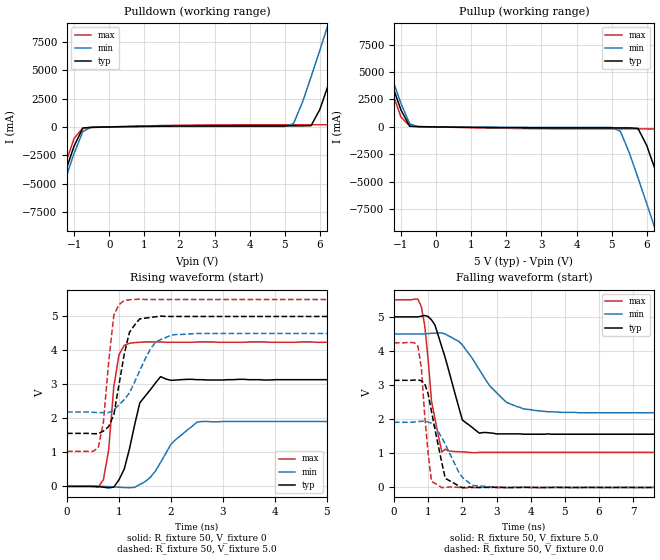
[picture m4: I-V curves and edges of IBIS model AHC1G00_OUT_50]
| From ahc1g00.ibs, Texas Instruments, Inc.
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|   Model AHC1G00_OUT_50
[Model]   AHC1G00_OUT_50
Model_type  Output
Polarity   Inverting
Vmeas = 2.50v
Cref = 15pf
| variable   typ   min   max
C_comp   3.12pf   2.34pf   3.90pf
[Temperature Range]   25   85   -40
[Voltage Range]   5.0   4.5   5.5
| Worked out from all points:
|   slope of the pulldown table from 0 to 0.75 V, typ, clamps not added: 18.8 ohm
|   slope of the pullup table from 0 to 0.75 V, typ, clamps not added: 25.3 ohm
|   rising waveform, R_fixture 50, V_fixture 0: 20-80 % time 307ps typ, 550ps min, 174ps max; typ from 0 V to 3.14 V
|   falling waveform, R_fixture 50, V_fixture 5.0: 20-80 % time 586ps typ, 1.03ns min, 304ps max; typ from 5 V to 1.56 V
|   rising waveform, R_fixture 50, V_fixture 5.0: 20-80 % time 250ps typ, 453ps min, 167ps max; typ from 1.56 V to 5 V
|   falling waveform, R_fixture 50, V_fixture 0.0: 20-80 % time 378ps typ, 581ps min, 209ps max; typ from 3.14 V to 0 V
[Pulldown]
|   Voltage   I(typ)   I(min)   I(max)
-5V       -40.9A     -41.4A     -40.3A
-1.75V    -8.76A     -9.39A     -8.09A
-1V       -1.69A     -2.33A     -1.02A
-750mV    -95.5mA    -395mA     -80.6mA
5.25V     93.4mA     298mA      192mA
5.75V     116mA      4.42A      192mA
6.25V     3.8A       9.19A      193mA
6.5V      6.17A      11.6A      931mA
6.75V     8.59A      14.1A      3.15A
7.25V     13.5A      19A        7.96A
7.5V      15.9A      21.4A      10.4A
10V       40.7A      46.2A      35.2A
[Pullup]
|   Voltage   I(typ)   I(min)   I(max)
-5V       40.7A      41.2A      40.1A
-2V       11A        11.6A      10.4A
-1.75V    8.59A      9.19A      7.96A
-1V       1.54A      2.14A      907mA
-750mV    63.6mA     284mA      62.5mA
5.25V     -84.4mA    -401mA     -178mA
5.75V     -130mA     -4.62A     -178mA
6.25V     -3.97A     -9.39A     -187mA
6.75V     -8.76A     -14.3A     -3.28A
7.25V     -13.6A     -19.2A     -8.09A
7.5V      -16.1A     -21.6A     -10.5A
10V       -40.9A     -46.4A     -35.3A
[Ramp]
| variable   typ   min   max
dV/dt_r   1.90E+00/3.24E-10   1.17E+00/4.90E-10   2.56E+00/1.49E-10
dV/dt_f   2.09E+00/5.17E-10   1.41E+00/1.00E-09   2.74E+00/2.95E-10
R_load = 50
[Rising Waveform]
R_fixture = 50
V_fixture = 0
|   Time   V(typ)   V(min)   V(max)
0s        0V         0V         0V
700ps     -23.1mV    -236uV     201mV
800ps     -43.2mV    -5.91mV    1.07V
900ps     -22.1mV    -13.9mV    2.94V
1ns       197mV      -24.2mV    3.88V
1.3ns     1.81V      -28.1mV    4.23V
1.4ns     2.46V      55.2mV     4.24V
1.8ns     3.23V      706mV      4.25V
2.6ns     3.14V      1.91V      4.25V
25ns      3.14V      1.91V      4.24V
[Falling Waveform]
R_fixture = 50
V_fixture = 5.0
V_fixture_min = 4.5
V_fixture_max = 5.5
|   Time   V(typ)   V(min)   V(max)
0s        5V         4.5V       5.5V
800ps     5.02V      4.5V       5.3V
900ps     5.04V      4.5V       4.75V
1.1ns     4.91V      4.52V      2.52V
1.4ns     4.12V      4.53V      1.04V
2ns       1.98V      4.18V      1.04V
2.5ns     1.59V      3.45V      1.03V
3.3ns     1.57V      2.49V      1.03V
4.5ns     1.57V      2.22V      1.03V
25ns      1.56V      2.19V      1.03V
[Rising Waveform]
R_fixture = 50
V_fixture = 5.0
V_fixture_min = 4.5
V_fixture_max = 5.5
|   Time   V(typ)   V(min)   V(max)
0s        1.56V      2.19V      1.03V
600ps     1.55V      2.17V      1.14V
700ps     1.63V      2.17V      1.9V
800ps     1.76V      2.17V      3.66V
900ps     2.11V      2.25V      5.04V
1.2ns     4.53V      2.75V      5.49V
1.4ns     4.93V      3.41V      5.51V
1.7ns     4.99V      4.24V      5.5V
2.5ns     5V         4.5V       5.5V
25ns      5V         4.5V       5.5V
[Falling Waveform]
R_fixture = 50
V_fixture = 0.0
|   Time   V(typ)   V(min)   V(max)
0s        3.14V      1.91V      4.24V
700ps     3.15V      1.93V      4.14V
800ps     3.13V      1.94V      3.53V
900ps     3.04V      1.94V      2.11V
1.1ns     2.22V      1.88V      173mV
1.4ns     728mV      1.46V      -7.56mV
1.5ns     269mV      1.27V      2.65mV
2ns       -9.68mV    301mV      -5.36mV
2.8ns     3.14mV     23.8mV     2.99mV
25ns      0V         0V         0V
